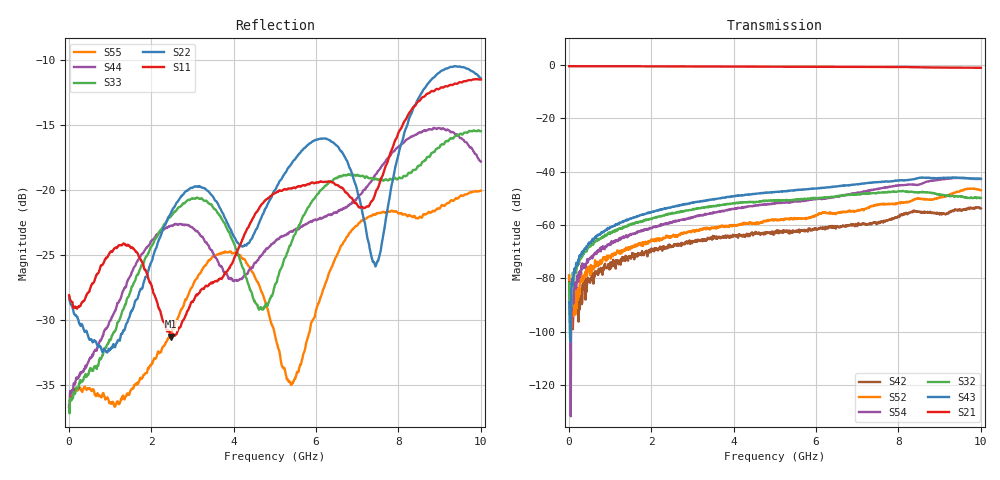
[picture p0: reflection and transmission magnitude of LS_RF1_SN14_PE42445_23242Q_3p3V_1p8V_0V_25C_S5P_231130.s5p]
!Keysight Technologies,M9804A,MY58100185,A.15.10.06
!Date: Thursday, November 30, 2023 12:04:16
!Correction: S11(Cdelta 6-Port  )
!S12(Cdelta 6-Port  )
!S13(Cdelta 6-Port  )
!S15(Cdelta 6-Port  )
!S16(Cdelta 6-Port  )
!S21(Cdelta 6-Port  )
!S22(Cdelta 6-Port  )
!S23(Cdelta 6-Port  )
!S25(Cdelta 6-Port  )
!S26(Cdelta 6-Port  )
!S31(Cdelta 6-Port  )
!S32(Cdelta 6-Port  )
!S33(Cdelta 6-Port  )
!S35(Cdelta 6-Port  )
!S36(Cdelta 6-Port  )
!S51(Cdelta 6-Port  )
!S52(Cdelta 6-Port  )
!S53(Cdelta 6-Port  )
!S55(Cdelta 6-Port  )
!S56(Cdelta 6-Port  )
!S61(Cdelta 6-Port  )
!S62(Cdelta 6-Port  )
!S63(Cdelta 6-Port  )
!S65(Cdelta 6-Port  )
!S66(Cdelta 6-Port  )
!S5P File: Measurements: <S11,S12,S13,S15,S16>,
!<S21,S22,S23,S25,S26>,
!<S31,S32,S33,S35,S36>,
!<S51,S52,S53,S55,S56>,
!<S61,S62,S63,S65,S66>:
# Hz S  dB  R 50
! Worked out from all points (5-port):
!   1000 points, 10 MHz to 10 GHz, reference 50 ohm
!   strongest paths, dB at 10 MHz, 2.51 GHz, 5.01 GHz, 7.51 GHz, 10 GHz:
!     S21: -0.6, -0.6, -0.7, -0.8, -1.1
!     S43: -89.0, -53.3, -47.6, -43.9, -42.7
!     S32: -81.7, -55.5, -50.9, -48.0, -49.9
!     S54: -91.3, -59.2, -52.0, -46.5, -42.8
!     S52: -79.1, -64.1, -58.1, -52.5, -47.0
!     S42: -79.0, -67.9, -63.1, -59.3, -53.8
!   lowest |S11| = -31.3 dB at 2.49 GHz (marker M1), VSWR 1.06, Z = 48.5 - j2.23 ohm
!   |S11| at or under -10 dB: start of sweep to end of sweep
